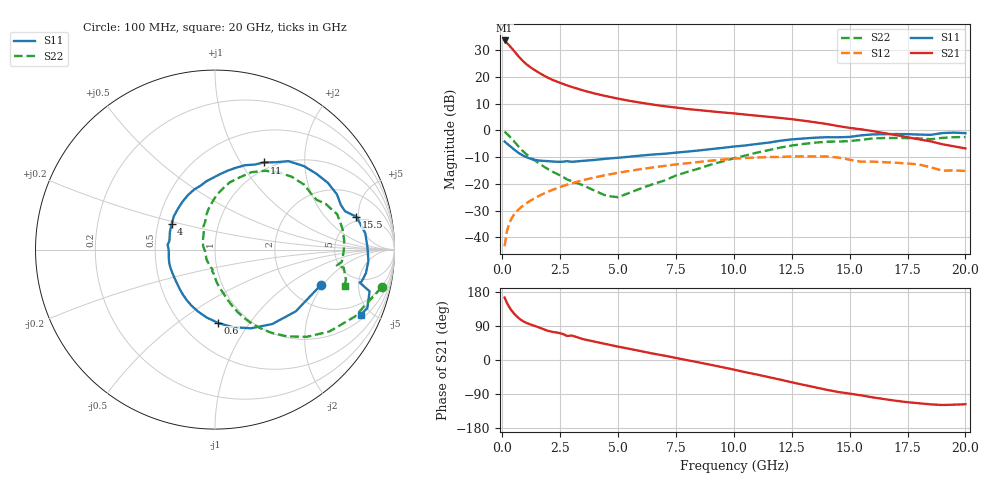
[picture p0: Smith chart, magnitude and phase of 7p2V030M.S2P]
! Infineon Technologies  Discrete & RF Semiconductors
! bfp620
! VCE =  2.0 V,  IC =  30 mA
! Common Emitter S-Parameters:  Sep 2002
# GHz  S  MA  R  50
!  f  S11  S21  S12  S22
! GHz  MAG  ANG  MAG  ANG  MAG  ANG  MAG  ANG
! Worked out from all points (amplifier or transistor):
!   59 points, 100 MHz to 20 GHz, reference 50 ohm
!   highest |S21| = 33.7 dB at 100 MHz (marker M1)
!   |S21| within 3 dB of that: start of sweep to 415.9 MHz
!   unconditionally stable (mu >= 1): 2.954 GHz to 9.874 GHz; 17.18 GHz to end of sweep
!   at 1 GHz: K = 0.77, MSG = 26.3 dB, |S12| = -27.5 dB
!   at 5.5 GHz: K = 1.04, MAG = 11.9 dB, |S12| = -15.1 dB
!   at 20 GHz: K = 1.28, MAG = 1.1 dB, |S12| = -15.2 dB
!   S11 on the Smith chart (normalised r, x): 100 MHz: 2.94, -1.90; 600 MHz: 0.74, -0.72; 4 GHz: 0.59, +0.18; 11 GHz: 0.90, +1.27; 15.5 GHz: 4.40, +4.66; 20 GHz: 1.25, -4.34
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0.1  0.6209 -18.7  48.38 164.8  0.0068 73.7  0.9513 -12.8
0.2  0.5668 -37.3  43.36 150.8  0.0129 70.4  0.8638 -25.6
0.3  0.5233 -52.4  39.02 139.7  0.0181 67.7  0.7839 -35.6
0.4  0.4821 -65.4  34.9 130.7  0.0225 65.5  0.7058 -43.5
0.5  0.4436 -77.0  31.03 123.1  0.0263 63.8  0.6309 -50.1
0.6  0.4095 -87.5  27.52 116.6  0.0298 62.4  0.5621 -55.7
0.7  0.3807 -97.1  24.47 111.0  0.033 61.4  0.5015 -60.4
0.9  0.3377 -113.1  19.77 102.3  0.0391 60.1  0.4066 -67.5
1.1  0.3083 -125.3  16.6 96.4  0.045 59.4  0.341 -72.1
1.3  0.2883 -135.2  14.39 92.0  0.0508 58.7  0.294 -75.4
1.8  0.2684 -156.7  10.63 80.8  0.0659 56.5  0.2099 -83.5
2.2  0.2615 -170.1  8.732 73.8  0.078 54.1  0.1662 -88.7
2.8  0.2655 174.1  6.955 63.5  0.0963 49.8  0.1207 -97.8
3.5  0.2695 158.9  5.595 54.8  0.1175 44.0  0.0934 -108.8
4  0.2804 149.8  4.897 48.3  0.1321 39.6  0.0739 -128.9
7  0.3654 102.7  2.841 11.5  0.2166 11.7  0.1151 123.0
10.5  0.5227 65.0  1.98 -32.2  0.3046 -27.3  0.3392 83.2
11  0.5575 60.6  1.886 -38.3  0.3108 -32.8  0.3842 77.5
13.5  0.7307 30.6  1.423 -71.9  0.325 -63.4  0.5894 43.5
15.5  0.8086 13.1  1.048 -93.3  0.2591 -85.5  0.6662 22.6
17  0.857 -4.2  0.82 -107.6  0.2476 -95.3  0.7215 3.8
20  0.8895 -24.1  0.46 -116.8  0.1741 -105.2  0.7512 -15.7
